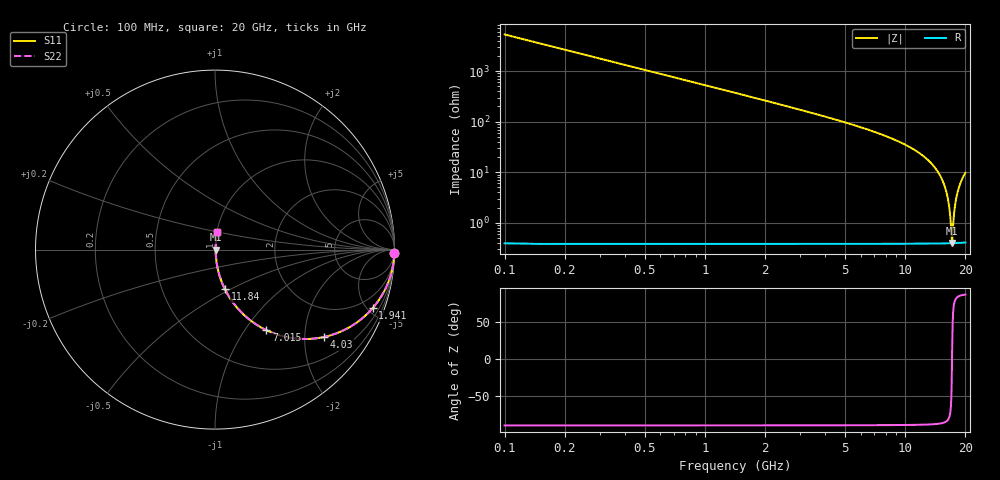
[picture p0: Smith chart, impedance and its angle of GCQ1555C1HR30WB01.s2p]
!Murata Part Number: GCQ1555C1HR30WB01
!These Parameters are Measured in Series Mode Connection
!Data Generated on Mar 13, 2026
!  o--ll--o
!Port1  Port2
!  o------o
!Operation Temp=25[degC], DC Bias Voltage=0[V]
!Freq. Start=100[MHz] Stop=20[GHz] 401[Steps]
# Hz S RI R 50
!Freq.(Hz) S11(Real) S11(Imag) S21(Real) S21(Imag) S12(Real) S12(Imag) S22(Real) S22(Imag)
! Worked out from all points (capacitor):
!   401 points, 100 MHz to 20 GHz, reference 50 ohm
!   read as one part in series: C = 300 fF near 199.5 MHz
!   lowest |Z| = 398 mohm at 17.16 GHz (marker M1)
!   series resonance near 17.15 GHz, so ESL is about 290 pH
!   S11 on the Smith chart (normalised r, x): 100 MHz: open; 1.941 GHz: 1.01, -5.40; 4.03 GHz: 1.01, -2.49; 7.015 GHz: 1.01, -1.26; 11.84 GHz: 1.01, -0.47; 20 GHz: 1.01, +0.19
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1e8  0.9996 -0.0188  0.000357 0.0188  0.000357 0.0188  0.9996 -0.0188
3.4875e8  0.9957 -0.0655  0.00432 0.0655  0.00432 0.0655  0.9957 -0.0655
6.97e8  0.9829 -0.1293  0.0171 0.1293  0.0171 0.1293  0.9829 -0.1293
1.1945e9  0.9511 -0.2151  0.0489 0.2151  0.0489 0.2151  0.9511 -0.2151
1.94075e9  0.8789 -0.3255  0.1211 0.3255  0.1211 0.3255  0.8789 -0.3255
3.43325e9  0.6872 -0.4623  0.3128 0.4623  0.3128 0.4623  0.6872 -0.4623
4.03025e9  0.6072 -0.4868  0.3928 0.4868  0.3928 0.4868  0.6072 -0.4868
6.7665e9  0.3063 -0.4581  0.6937 0.4581  0.6937 0.4581  0.3063 -0.4581
7.01525e9  0.2857 -0.4487  0.7143 0.4487  0.7143 0.4487  0.2857 -0.4487
1.005e10  0.1106 -0.3081  0.8894 0.3081  0.8894 0.3081  0.1106 -0.3081
1.1841e10  0.0559 -0.2216  0.9441 0.2216  0.9441 0.2216  0.0559 -0.2216
1.338325e10  0.0274 -0.1512  0.9726 0.1512  0.9726 0.1512  0.0274 -0.1512
1.467675e10  0.0132 -0.0959  0.9868 0.0959  0.9868 0.0959  0.0132 -0.0959
1.5622e10  0.00726 -0.0578  0.9927 0.0578  0.9927 0.0578  0.00726 -0.0578
1.626875e10  0.00499 -0.0328  0.995 0.0328  0.995 0.0328  0.00499 -0.0328
1.67165e10  0.00418 -0.0159  0.9958 0.0159  0.9958 0.0159  0.00418 -0.0159
1.706475e10  0.00394 -0.00314  0.9961 0.00314  0.9961 0.00314  0.00394 -0.00314
1.716425e10  0.00394 0.000473  0.9961 -0.000473  0.9961 -0.000473  0.00394 0.000473
1.7612e10  0.00422 0.0165  0.9958 -0.0165  0.9958 -0.0165  0.00422 0.0165
1.805975e10  0.005 0.0321  0.995 -0.0321  0.995 -0.0321  0.005 0.0321
1.885575e10  0.00751 0.059  0.9925 -0.059  0.9925 -0.059  0.00751 0.059
2e10  0.0134 0.0958  0.9866 -0.0958  0.9866 -0.0958  0.0134 0.0958
